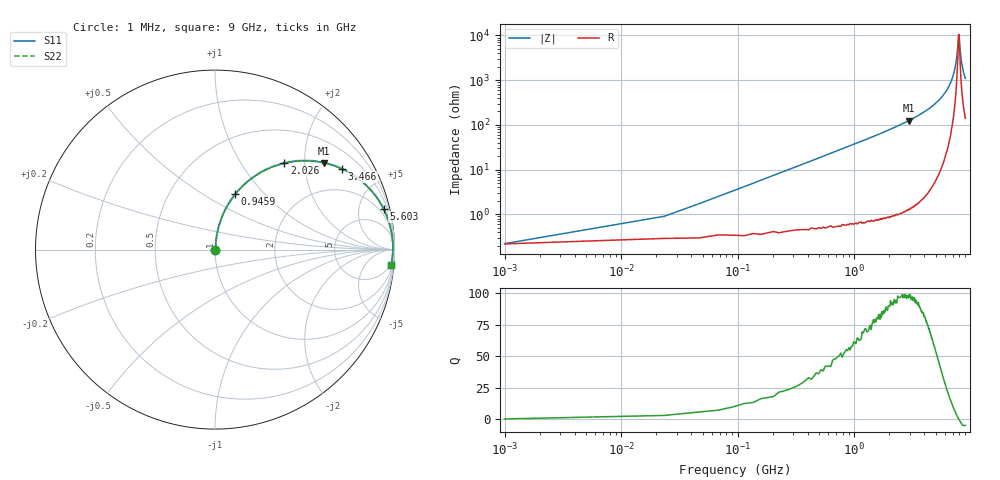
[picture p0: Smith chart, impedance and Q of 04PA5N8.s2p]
! Coilcraft 0402PA-5N8 Chip Inductor
! 11 March 2004
# MHZ S MA R 50
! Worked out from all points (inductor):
!   401 points, 1 MHz to 9 GHz, reference 50 ohm
!   read as one part in series: L = 5.79 nH near 45.99 MHz
!   highest Q = 97.8 at 2.948 GHz (marker M1), where L = 6.74 nH
!   self-resonance near 7.898 GHz
!   S11 on the Smith chart (normalised r, x): 1 MHz: 1.00, +0.00; 945.9 MHz: 1.01, +0.70; 2.026 GHz: 1.02, +1.58; 3.466 GHz: 1.04, +3.13; 5.603 GHz: 1.21, +8.21; 9 GHz: 4, -22
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1  0.002363 8.8  0.998 -0.0  0.998 -0.0  0.002363 8.8
68.492  0.025 81.2  0.996 -1.4  0.996 -1.4  0.025 81.2
90.99  0.033 82.3  0.996 -1.9  0.996 -1.9  0.033 82.3
158.482  0.058 83.0  0.995 -3.3  0.995 -3.3  0.058 83.0
225.975  0.082 82.5  0.993 -4.7  0.993 -4.7  0.082 82.5
495.945  0.178 78.2  0.979 -10.2  0.979 -10.2  0.178 78.2
945.895  0.328 69.8  0.939 -19.2  0.939 -19.2  0.328 69.8
1508.332  0.493 59.7  0.864 -29.5  0.864 -29.5  0.493 59.7
2025.775  0.617 51.3  0.78 -38.1  0.78 -38.1  0.617 51.3
2948.172  0.777 38.5  0.622 -50.9  0.622 -50.9  0.777 38.5
3015.665  0.786 37.6  0.611 -51.8  0.611 -51.8  0.786 37.6
3465.615  0.838 32.4  0.536 -57.0  0.536 -57.0  0.838 32.4
4500.5  0.92 22.3  0.379 -66.9  0.379 -66.9  0.92 22.3
5602.878  0.966 13.6  0.235 -74.9  0.235 -74.9  0.966 13.6
6007.833  0.976 10.8  0.188 -77.2  0.188 -77.2  0.976 10.8
6952.728  0.988 5.0  0.088 -79.9  0.088 -79.9  0.988 5.0
7515.165  0.991 2.0  0.036 -73.8  0.036 -73.8  0.991 2.0
7897.623  0.991 0.0  0.009403 -1.7  0.009403 -1.7  0.991 0.0
7965.115  0.99 -0.3  0.011 30.0  0.011 30.0  0.99 -0.3
8145.095  0.99 -1.2  0.023 63.6  0.023 63.6  0.99 -1.2
8347.573  0.989 -2.2  0.039 72.7  0.039 72.7  0.989 -2.2
9000  0.984 -5.1  0.09 77.5  0.09 77.5  0.984 -5.1
